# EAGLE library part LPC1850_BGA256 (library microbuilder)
LPC1850/LPC4350 - LBGA256 Warning: This footprint was designed for a specific application, and numerous choices have been made concering the PINMUX to make certain peripherals available at the expense of others. These pin choices may not be appropriate in your own situation (for example, only one set of selection pins is broken out for the EMC rather than all four, although some pins on GPIO6 can be sacrificed to enable another memory device on the EMC using CS2).
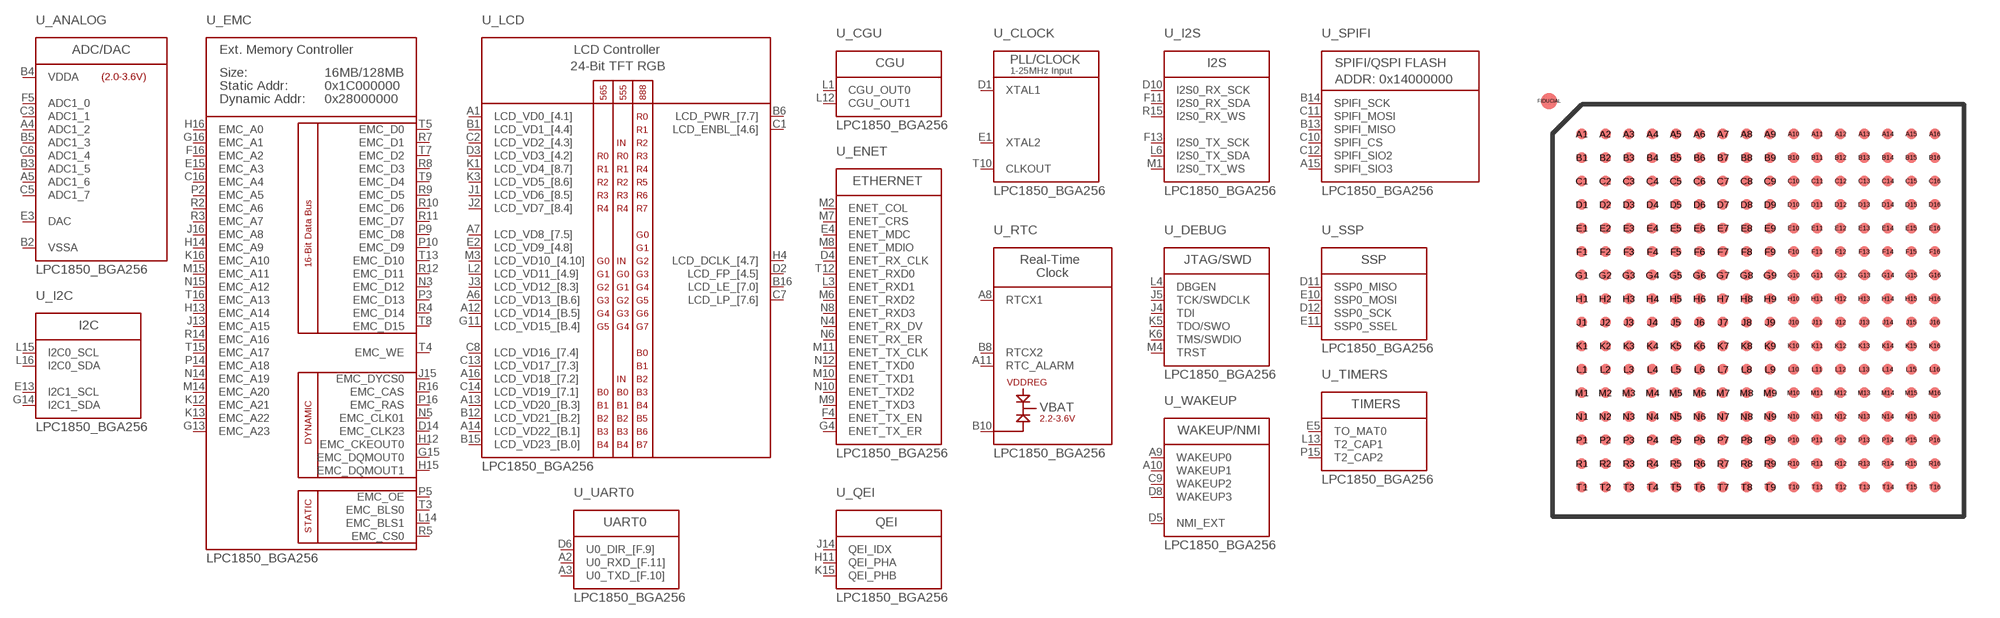
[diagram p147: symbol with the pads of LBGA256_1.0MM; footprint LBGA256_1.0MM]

Designator prefix U; gates _ANALOG=LPC1850_ADC _EMC=LPC1850_EMC _LCD=LPC1850_LCD _RTC=LPC1850_RTC _CGU=LPC1850_CGU _ENET=LPC1850_ETHERNET _CLOCK=LPC1850_CLOCK _I2C=LPC1850_I2C _I2S=LPC1850_I2S _DEBUG=LPC1850_JTAG _WAKEUP=LPC1850_NMI_WAKEUP _QEI=LPC1850_QEI _SPIFI=LPC1850_SPIFI _SSP=LPC1850_SSP _TIMERS=LPC1850_TIMERS _UART0=LPC1850_UART0 _UART1=LPC1850_UART1 _USB0_HS=LPC1850_USB0 _USB1=LPC1850_USB1 _GPIO=LPC1850_GPIO _GPIO6=LPC1850_GPIO6 _POWER=LPC1850_POWER _RESET=LPC1850_RESET

## LPC1850_BGA256  [LBGA256_1.0MM]
A1  _LCD:LCD_VD0_[4.1]
A2  _UART0:U0_RXD_[F.11]
A3  _UART0:U0_TXD_[F.10]
A4  _ANALOG:ADC1_2
A5  _ANALOG:ADC1_6
A6  _LCD:LCD_VD13_[B.6]
A7  _LCD:LCD_VD8_[7.5]
A8  _RTC:RTCX1
A9  _WAKEUP:WAKEUP0
A10  _WAKEUP:WAKEUP1
A11  _RTC:RTC_ALARM
A12  _LCD:LCD_VD14_[B.5]
A13  _LCD:LCD_VD20_[B.3]
A14  _LCD:LCD_VD22_[B.1]
A15  _SPIFI:SPIFI_SIO3
A16  _LCD:LCD_VD18_[7.2]
B1  _LCD:LCD_VD1_[4.4]
B2  _ANALOG:VSSA
B3  _ANALOG:ADC1_5
B4  _ANALOG:VDDA
B5  _ANALOG:ADC1_3
B6  _LCD:LCD_PWR_[7.7]
B7  _GPIO:GPIO7[21]
B8  _RTC:RTCX2
B10  _RTC:VBAT
B11  _GPIO:GPIO5[24]
B12  _LCD:LCD_VD21_[B.2]
B13  _SPIFI:SPIFI_MISO
B14  _SPIFI:SPIFI_SCK
B15  _LCD:LCD_VD23_[B.0]
B16  _LCD:LCD_LE_[7.0]
C1  _LCD:LCD_ENBL_[4.6]
C2  _LCD:LCD_VD2_[4.3]
C3  _ANALOG:ADC1_1
C4  _POWER:VSSIO  pwr
C5  _ANALOG:ADC1_7
C6  _ANALOG:ADC1_4
C7  _LCD:LCD_LP_[7.6]
C8  _LCD:LCD_VD16_[7.4]
C9  _WAKEUP:WAKEUP2
C10  _SPIFI:SPIFI_CS
C11  _SPIFI:SPIFI_MOSI
C12  _SPIFI:SPIFI_SIO2
C13  _LCD:LCD_VD17_[7.3]
C14  _LCD:LCD_VD19_[7.1]
C15  _GPIO:GPIO7[14]
C16  _EMC:EMC_A4
D1  _CLOCK:XTAL1
D2  _LCD:LCD_FP_[4.5]
D3  _LCD:LCD_VD3_[4.2]
D4  _ENET:ENET_RX_CLK
D5  _WAKEUP:NMI_EXT
D6  _UART0:U0_DIR_[F.9]
D7  _POWER:VDDIO  pwr
D8  _WAKEUP:WAKEUP3
D9  _RESET:RESET
D10  _I2S:I2S0_RX_SCK
D11  _SSP:SSP0_MISO
D12  _SSP:SSP0_SCK
D13  _POWER:VSSIO  pwr
D14  _EMC:EMC_CLK23
D15  _UART1:U1_RXD
D16  _UART1:U1_TXD
E1  _CLOCK:XTAL2
E2  _LCD:LCD_VD9_[4.8]
E3  _ANALOG:DAC
E4  _ENET:ENET_MDC
E5  _TIMERS:TO_MAT0
E6  _GPIO:GPIO7[22]
E7  _GPIO:GPIO7[20]
E8  _POWER:VPP  pwr
E9  _GPIO:GPIO7[19]
E10  _SSP:SSP0_MOSI
E11  _SSP:SSP0_SSEL
E12  _POWER:VDDIO  pwr
E13  _I2C:I2C1_SCL
E14  _UART1:U1_DTR
E15  _EMC:EMC_A3
E16  _UART1:U1_DCD
F1  _USB0_HS:USB0_VBUS
F2  _USB0_HS:USB0_DP
F3  _USB0_HS:USB0_VDDA3V3_DRIVER
F4  _ENET:ENET_TX_EN
F5  _ANALOG:ADC1_0
F6  _GPIO6:GPIO6[1]
F7  _POWER:VDDIO  pwr
F8  _POWER:VDDIO  pwr
F9  _POWER:VDDREG  pwr
F10  _POWER:VDDREG  pwr
F11  _I2S:I2S0_RX_SDA
F12  _USB1:USB1_DP
F13  _I2S:I2S0_TX_SCK
F14  _UART1:U1_DSR
F15  _UART1:U1_CTS
F16  _EMC:EMC_A2
G1  _USB0_HS:USB0_VSSA_REF
G2  _USB0_HS:USB0_DM
G3  _USB0_HS:USB0_VDDA3V3
G4  _ENET:ENET_TX_ER
G5  _GPIO6:GPIO6[6]
G6  _POWER:VSSIO  pwr
G7  _POWER:VSSIO  pwr
G8  _POWER:VSSIO  pwr
G9  _POWER:VSS  pwr
G10  _POWER:VDDIO  pwr
G11  _LCD:LCD_VD15_[B.4]
G12  _USB1:USB1_DM
G13  _EMC:EMC_A23
G14  _I2C:I2C1_SDA
G15  _EMC:EMC_DQMOUT0
G16  _EMC:EMC_A1
H1  _USB0_HS:USB0_RREF
H2  _USB0_HS:USB0_ID
H3  _USB0_HS:USB0_VSSA_TERM
H4  _LCD:LCD_DCLK_[4.7]
H5  _USB0_HS:USB0_IND1
H6  _GPIO6:GPIO6[5]
H7  _POWER:VSS  pwr
H8  _POWER:VSSIO  pwr
H9  _POWER:VSSIO  pwr
H10  _POWER:VDDIO  pwr
H11  _QEI:QEI_PHA
H12  _EMC:EMC_CKEOUT0
H13  _EMC:EMC_A14
H14  _EMC:EMC_A9
H15  _EMC:EMC_DQMOUT1
H16  _EMC:EMC_A0
J1  _LCD:LCD_VD6_[8.5]
J2  _LCD:LCD_VD7_[8.4]
J3  _LCD:LCD_VD12_[8.3]
J4  _DEBUG:TDI
J5  _DEBUG:TCK/SWDCLK
J6  _POWER:VDDIO  pwr
J7  _POWER:VDDIO  pwr
J8  _POWER:VSSIO  pwr
J9  _POWER:VSSIO  pwr
J10  _POWER:VSS  pwr
J11  _POWER:VSS  pwr
J12  _USB0_HS:USB0_PWR_EN
J13  _EMC:EMC_A15
J14  _QEI:QEI_IDX
J15  _EMC:EMC_DYCS0
J16  _EMC:EMC_A8
K1  _LCD:LCD_VD4_[8.7]
K2  _GPIO6:GPIO6[8]
K3  _LCD:LCD_VD5_[8.6]
K4  _USB0_HS:USB0_IND0
K5  _DEBUG:TDO/SWO
K6  _DEBUG:TMS/SWDIO
K7  _POWER:VDDIO  pwr
K8  _POWER:VSS  pwr
K9  _POWER:VSSIO  pwr
K10  _POWER:VSSIO  pwr
K11  _USB0_HS:USB0_PWR_FAULT
K12  _EMC:EMC_A21
K13  _EMC:EMC_A22
K14  _USB1:USB1_VBUS
K15  _QEI:QEI_PHB
K16  _EMC:EMC_A10
L1  _CGU:CGU_OUT0
L2  _LCD:LCD_VD11_[4.9]
L3  _ENET:ENET_RXD1
L4  _DEBUG:DBGEN
L5  _GPIO6:GPIO6[10]
L6  _I2S:I2S0_TX_SDA
L7  _POWER:VDDREG  pwr
L8  _POWER:VDDREG  pwr
L9  _POWER:VDDIO  pwr
L10  _POWER:VDDIO  pwr
L11  _GPIO:GPIO4[11]
L12  _CGU:CGU_OUT1
L13  _TIMERS:T2_CAP1
L14  _EMC:EMC_BLS1
L15  _I2C:I2C0_SCL
L16  _I2C:I2C0_SDA
M1  _I2S:I2S0_TX_WS
M2  _ENET:ENET_COL
M3  _LCD:LCD_VD10_[4.10]
M4  _DEBUG:TRST
M5  _GPIO6:GPIO6[9]
M6  _ENET:ENET_RXD2
M7  _ENET:ENET_CRS
M8  _ENET:ENET_MDIO
M9  _ENET:ENET_TXD3
M10  _ENET:ENET_TXD1
M11  _ENET:ENET_TX_CLK
M13  _POWER:VSSIO  pwr
M14  _EMC:EMC_A20
M15  _EMC:EMC_A11
M16  _UART1:U1_RI
N1  _GPIO6:GPIO6[13]
N2  _GPIO6:GPIO6[14]
N3  _EMC:EMC_D12
N4  _ENET:ENET_RX_DV
N5  _EMC:EMC_CLK01
N6  _ENET:ENET_RX_ER
N7  _POWER:VDDIO  pwr
N8  _ENET:ENET_RXD3
N9  _GPIO6:GPIO6[25]
N10  _ENET:ENET_TXD2
N11  _GPIO6:GPIO6[26]
N12  _ENET:ENET_TXD0
N13  _POWER:VDDIO  pwr
N14  _EMC:EMC_A19
N15  _EMC:EMC_A12
N16  _UART1:U1_RTS
P1  _GPIO6:GPIO6[15]
P2  _EMC:EMC_A5
P3  _EMC:EMC_D13
P4  _GPIO6:GPIO6[17]
P5  _EMC:EMC_OE
P6  _GPIO6:GPIO6[19]
P7  _POWER:VSSIO  pwr
P8  _GPIO6:GPIO6[22]
P9  _EMC:EMC_D8
P10  _EMC:EMC_D9
P11  _GPIO6:GPIO6[24]
P13  _POWER:VSSIO  pwr
P14  _EMC:EMC_A18
P15  _TIMERS:T2_CAP2
P16  _EMC:EMC_RAS
R1  _GPIO6:GPIO6[16]
R2  _EMC:EMC_A6
R3  _EMC:EMC_A7
R4  _EMC:EMC_D14
R5  _EMC:EMC_CS0
R6  _GPIO6:GPIO6[20]
R7  _EMC:EMC_D1
R8  _EMC:EMC_D3
R9  _EMC:EMC_D5
R10  _EMC:EMC_D6
R11  _EMC:EMC_D7
R12  _EMC:EMC_D11
R13  _GPIO6:GPIO6[28]
R14  _EMC:EMC_A16
R15  _I2S:I2S0_RX_WS
R16  _EMC:EMC_CAS
T1  _GPIO:GPIO4[12]
T2  _GPIO6:GPIO6[18]
T3  _EMC:EMC_BLS0
T4  _EMC:EMC_WE
T5  _EMC:EMC_D0
T6  _GPIO6:GPIO6[21]
T7  _EMC:EMC_D2
T8  _EMC:EMC_D15
T9  _EMC:EMC_D4
T10  _CLOCK:CLKOUT
T11  _GPIO6:GPIO6[23]
T12  _ENET:ENET_RXD0
T13  _EMC:EMC_D10
T14  _GPIO6:GPIO6[27]
T15  _EMC:EMC_A17
T16  _EMC:EMC_A13

## Footprint LBGA256_1.0MM (pad centres in mm)
LBGA256 - SOT740-2 LBGA256: plastic low profile ball grid array package; 256 balls; body 17 x 17 x 1 mm
smd 0.45 x 0.45: A1 -7.5,7.5; A2 -6.5,7.5; A3 -5.5,7.5; A4 -4.5,7.5; A5 -3.5,7.5; A6 -2.5,7.5; A7 -1.5,7.5; A8 -0.5,7.5; A9 0.5,7.5; A10 1.5,7.5; A11 2.5,7.5; A12 3.5,7.5; A13 4.5,7.5; A14 5.5,7.5; A15 6.5,7.5; A16 7.5,7.5; B1 -7.5,6.5; B2 -6.5,6.5; B3 -5.5,6.5; B4 -4.5,6.5; B5 -3.5,6.5; B6 -2.5,6.5; B7 -1.5,6.5; B8 -0.5,6.5; B9 0.5,6.5; B10 1.5,6.5; B11 2.5,6.5; B12 3.5,6.5; B13 4.5,6.5; B14 5.5,6.5; B15 6.5,6.5; B16 7.5,6.5; C1 -7.5,5.5; C2 -6.5,5.5; C3 -5.5,5.5; C4 -4.5,5.5; C5 -3.5,5.5; C6 -2.5,5.5; C7 -1.5,5.5; C8 -0.5,5.5; C9 0.5,5.5; C10 1.5,5.5; C11 2.5,5.5; C12 3.5,5.5; C13 4.5,5.5; C14 5.5,5.5; C15 6.5,5.5; C16 7.5,5.5; D1 -7.5,4.5; D2 -6.5,4.5; D3 -5.5,4.5; D4 -4.5,4.5; D5 -3.5,4.5; D6 -2.5,4.5; D7 -1.5,4.5; D8 -0.5,4.5; D9 0.5,4.5; D10 1.5,4.5; D11 2.5,4.5; D12 3.5,4.5; D13 4.5,4.5; D14 5.5,4.5; D15 6.5,4.5; D16 7.5,4.5; E1 -7.5,3.5; E2 -6.5,3.5; E3 -5.5,3.5; E4 -4.5,3.5; E5 -3.5,3.5; E6 -2.5,3.5; E7 -1.5,3.5; E8 -0.5,3.5; E9 0.5,3.5; E10 1.5,3.5; E11 2.5,3.5; E12 3.5,3.5; E13 4.5,3.5; E14 5.5,3.5; E15 6.5,3.5; E16 7.5,3.5; F1 -7.5,2.5; F2 -6.5,2.5; F3 -5.5,2.5; F4 -4.5,2.5; F5 -3.5,2.5; F6 -2.5,2.5; F7 -1.5,2.5; F8 -0.5,2.5; F9 0.5,2.5; F10 1.5,2.5; F11 2.5,2.5; F12 3.5,2.5; F13 4.5,2.5; F14 5.5,2.5; F15 6.5,2.5; F16 7.5,2.5; G1 -7.5,1.5; G2 -6.5,1.5; G3 -5.5,1.5; G4 -4.5,1.5; G5 -3.5,1.5; G6 -2.5,1.5; G7 -1.5,1.5; G8 -0.5,1.5; G9 0.5,1.5; G10 1.5,1.5; G11 2.5,1.5; G12 3.5,1.5; G13 4.5,1.5; G14 5.5,1.5; G15 6.5,1.5; G16 7.5,1.5; H1 -7.5,0.5; H2 -6.5,0.5; H3 -5.5,0.5; H4 -4.5,0.5; H5 -3.5,0.5; H6 -2.5,0.5; H7 -1.5,0.5; H8 -0.5,0.5; H9 0.5,0.5; H10 1.5,0.5; H11 2.5,0.5; H12 3.5,0.5; H13 4.5,0.5; H14 5.5,0.5; H15 6.5,0.5; H16 7.5,0.5; J1 -7.5,-0.5; J2 -6.5,-0.5; J3 -5.5,-0.5; J4 -4.5,-0.5; J5 -3.5,-0.5; J6 -2.5,-0.5; J7 -1.5,-0.5; J8 -0.5,-0.5; J9 0.5,-0.5; J10 1.5,-0.5; J11 2.5,-0.5; J12 3.5,-0.5; J13 4.5,-0.5; J14 5.5,-0.5; J15 6.5,-0.5; J16 7.5,-0.5; K1 -7.5,-1.5; K2 -6.5,-1.5; K3 -5.5,-1.5; K4 -4.5,-1.5; K5 -3.5,-1.5; K6 -2.5,-1.5; K7 -1.5,-1.5; K8 -0.5,-1.5; K9 0.5,-1.5; K10 1.5,-1.5; K11 2.5,-1.5; K12 3.5,-1.5; K13 4.5,-1.5; K14 5.5,-1.5; K15 6.5,-1.5; K16 7.5,-1.5; L1 -7.5,-2.5; L2 -6.5,-2.5; L3 -5.5,-2.5; L4 -4.5,-2.5; L5 -3.5,-2.5; L6 -2.5,-2.5; L7 -1.5,-2.5; L8 -0.5,-2.5; L9 0.5,-2.5; L10 1.5,-2.5; L11 2.5,-2.5; L12 3.5,-2.5; L13 4.5,-2.5; L14 5.5,-2.5; L15 6.5,-2.5; L16 7.5,-2.5; M1 -7.5,-3.5; M2 -6.5,-3.5; M3 -5.5,-3.5; M4 -4.5,-3.5; M5 -3.5,-3.5; M6 -2.5,-3.5; M7 -1.5,-3.5; M8 -0.5,-3.5; M9 0.5,-3.5; M10 1.5,-3.5; M11 2.5,-3.5; M12 3.5,-3.5; M13 4.5,-3.5; M14 5.5,-3.5; M15 6.5,-3.5; M16 7.5,-3.5; N1 -7.5,-4.5; N2 -6.5,-4.5; N3 -5.5,-4.5; N4 -4.5,-4.5; N5 -3.5,-4.5; N6 -2.5,-4.5; N7 -1.5,-4.5; N8 -0.5,-4.5; N9 0.5,-4.5; N10 1.5,-4.5; N11 2.5,-4.5; N12 3.5,-4.5; N13 4.5,-4.5; N14 5.5,-4.5; N15 6.5,-4.5; N16 7.5,-4.5; P1 -7.5,-5.5; P2 -6.5,-5.5; P3 -5.5,-5.5; P4 -4.5,-5.5; P5 -3.5,-5.5; P6 -2.5,-5.5; P7 -1.5,-5.5; P8 -0.5,-5.5; P9 0.5,-5.5; P10 1.5,-5.5; P11 2.5,-5.5; P12 3.5,-5.5; P13 4.5,-5.5; P14 5.5,-5.5; P15 6.5,-5.5; P16 7.5,-5.5; R1 -7.5,-6.5; R2 -6.5,-6.5; R3 -5.5,-6.5; R4 -4.5,-6.5; R5 -3.5,-6.5; R6 -2.5,-6.5; R7 -1.5,-6.5; R8 -0.5,-6.5; R9 0.5,-6.5; R10 1.5,-6.5; R11 2.5,-6.5; R12 3.5,-6.5; R13 4.5,-6.5; R14 5.5,-6.5; R15 6.5,-6.5; R16 7.5,-6.5; T1 -7.5,-7.5; T2 -6.5,-7.5; T3 -5.5,-7.5; T4 -4.5,-7.5; T5 -3.5,-7.5; T6 -2.5,-7.5; T7 -1.5,-7.5; T8 -0.5,-7.5; T9 0.5,-7.5; T10 1.5,-7.5; T11 2.5,-7.5; T12 3.5,-7.5; T13 4.5,-7.5; T14 5.5,-7.5; T15 6.5,-7.5; T16 7.5,-7.5
smd 0.7 x 0.7: FIDUCIAL -8.89,8.89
